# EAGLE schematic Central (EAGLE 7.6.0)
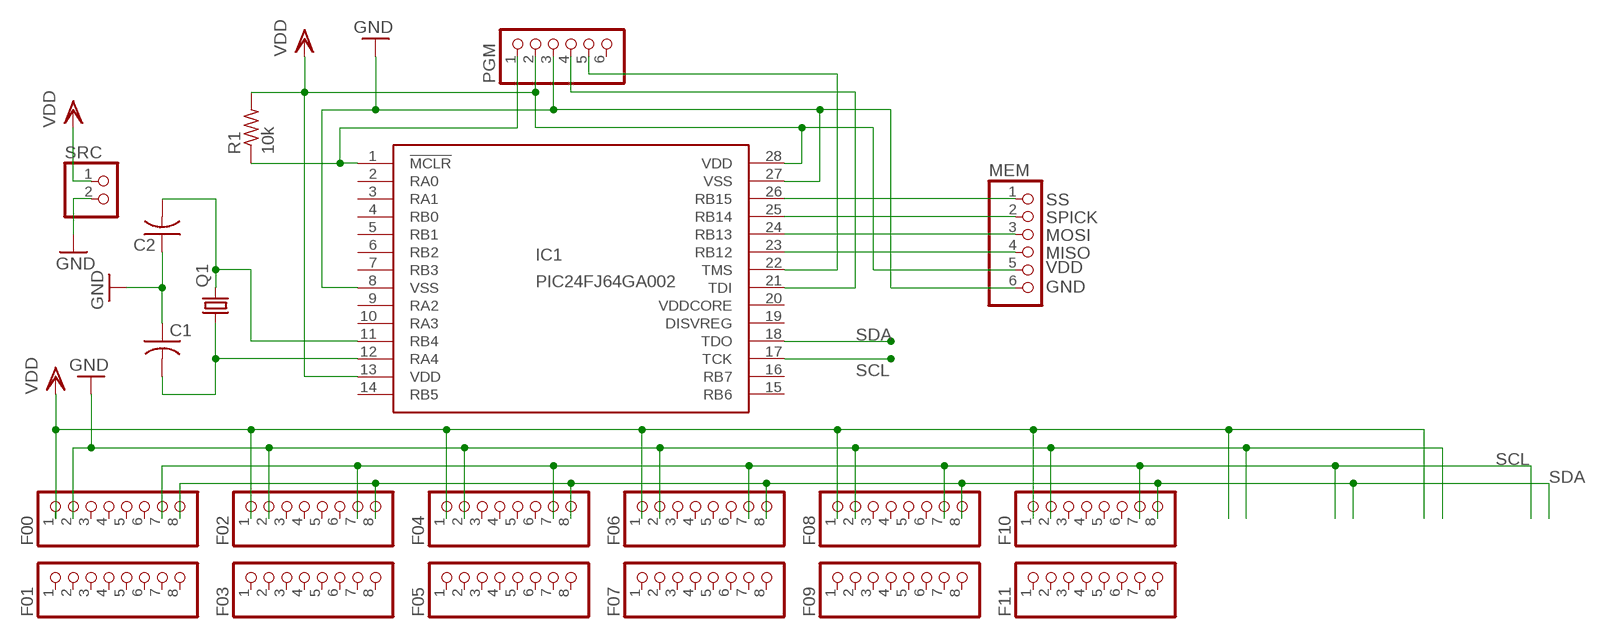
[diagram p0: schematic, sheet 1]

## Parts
C1  C-US025-030X050  [C025-030X050]
C2  C-US025-030X050  [C025-030X050]
F00  PINHD-1X8  [1X08]
F01  PINHD-1X8  [1X08]
F02  PINHD-1X8  [1X08]
F03  PINHD-1X8  [1X08]
F04  PINHD-1X8  [1X08]
F05  PINHD-1X8  [1X08]
F06  PINHD-1X8  [1X08]
F07  PINHD-1X8  [1X08]
F08  PINHD-1X8  [1X08]
F09  PINHD-1X8  [1X08]
F10  PINHD-1X8  [1X08]
F11  PINHD-1X8  [1X08]
IC1  PIC24FJ64GA002  [DIL28-3]
MEM  PINHD-1X6  [1X06]
PGM  PINHD-1X6  [1X06]
Q1  CRYSTALTC26V  [TC26V]
R1  10k  R-US_0204/7  [0204/7]
SRC  PINHD-1X2  [1X02]

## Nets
GND: C1.1 C2.1 F00.2 F02.2 F04.2 F06.2 F08.2 F10.2 IC1.8(VSS) IC1.27(VSS) MEM.6 PGM.3 SRC.2
MISO: IC1.23(RB12) MEM.4
MOSI: IC1.24(RB13) MEM.3
N$1: IC1.1(!MCLR) PGM.1 R1.1
N$2: C1.2 IC1.12(RA4) Q1.1
N$3: C2.2 IC1.11(RB4) Q1.2
N$4: IC1.21(TDI) PGM.4
N$5: IC1.22(TMS) PGM.5
SCL: F00.7 F02.7 F04.7 F06.7 F08.7 F10.7 IC1.17(TCK)
SDA: F00.8 F02.8 F04.8 F06.8 F08.8 F10.8 IC1.18(TDO)
SPICK: IC1.25(RB14) MEM.2
SS: IC1.26(RB15) MEM.1
VDD: F00.1 F02.1 F04.1 F06.1 F08.1 F10.1 IC1.13(VDD) IC1.28(VDD) MEM.5 PGM.2 R1.2 SRC.1
Unconnected: F00.3 F00.4 F00.5 F00.6 F01.1 F01.2 F01.3 F01.4 F01.5 F01.6 F01.7 F01.8 F02.3 F02.4 F02.5 F02.6 F03.1 F03.2 F03.3 F03.4 F03.5 F03.6 F03.7 F03.8 F04.3 F04.4 F04.5 F04.6 F05.1 F05.2 F05.3 F05.4 F05.5 F05.6 F05.7 F05.8 F06.3 F06.4 F06.5 F06.6 F07.1 F07.2 F07.3 F07.4 F07.5 F07.6 F07.7 F07.8 F08.3 F08.4 F08.5 F08.6 F09.1 F09.2 F09.3 F09.4 F09.5 F09.6 F09.7 F09.8 F10.3 F10.4 F10.5 F10.6 F11.1 F11.2 F11.3 F11.4 F11.5 F11.6 F11.7 F11.8 IC1.2(RA0) IC1.3(RA1) IC1.4(RB0) IC1.5(RB1) IC1.6(RB2) IC1.7(RB3) IC1.9(RA2) IC1.10(RA3) IC1.14(RB5) IC1.15(RB6) IC1.16(RB7) IC1.19(DISVREG) PGM.6

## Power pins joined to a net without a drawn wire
VDDCORE: IC1.20(VDDCORE)

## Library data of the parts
C1 C2 = adafruit:C-US: CAPACITOR, American symbol
F00 F01-F09 F10 F11 = pinhead:PINHD-1X8: PIN HEADER
IC1 = microchip:PIC24FJ64GA002: PIC24FJ64GA002 edit this description Auto generated by make-symbol-device-package-bsdl.ulp Rev. 25 Source: PIC24FJ64GA002.bsd; MPN: PIC24FJ64GA002-I/SP; OC_FARNELL: 1332298; OC_NEWARK: 88K6132
MEM PGM = pinhead:PINHD-1X6: PIN HEADER
Q1 = crystal:CRYSTAL: CRYSTAL; OC_FARNELL: unknown; OC_NEWARK: unknown
R1 = resistor:R-US_: RESISTOR, American symbol
SRC = pinhead:PINHD-1X2: PIN HEADER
